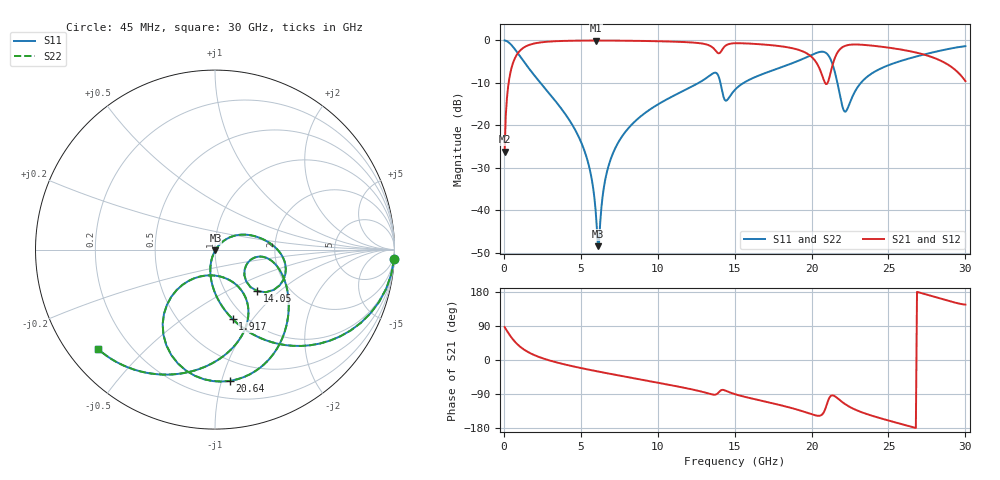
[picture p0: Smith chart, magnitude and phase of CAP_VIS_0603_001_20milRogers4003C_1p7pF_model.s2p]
! S-parameter model data by Modelithics Inc.  support@modelithics.com  813-866-6335  Tampa FL USA
! S-Parameter data specifications:
! Substrate: 20-mil Rogers 4003C, substrate thickness, H=0.508mm, Dielectric constant, Er=3.75
! PCB Mounting Pad Footprint: Pad width, PadW=0.90mm , Pad length, PadL=1.00mm , Pad gap, PadG (edge-to-edge)=1.00mm , Reference planes=3.0mm apart
! Created Wed Nov 18 13:18:57 2015
# hz S ma R 50
! 2 Port Network Data from SP1.SP block
! freq  magS11  angS11  magS21  angS21  magS12  angS12  magS22  angS22
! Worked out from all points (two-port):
!   401 points, 45 MHz to 30 GHz, reference 50 ohm
!   highest |S21| = -0.03 dB at 5.961 GHz (marker M1); lowest = -26.2 dB at 45 MHz (marker M2)
!   |S21| within 3 dB of the highest: 902.1 MHz to 13.95 GHz (13.05 GHz wide, 176 % of centre); 13.99 GHz to 19.68 GHz (5.691 GHz wide, 33.8 % of centre)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
!   lowest |S11| = -48.5 dB at 6.111 GHz (marker M3), VSWR 1.01, Z = 50.2 - j0.303 ohm
!   |S11| at or under -10 dB: 2.372 GHz to 12.67 GHz (10.29 GHz wide, 137 % of centre); 14.07 GHz to 15.59 GHz (1.516 GHz wide, 10.2 % of centre); 21.68 GHz to 23.21 GHz (1.529 GHz wide, 6.81 % of centre)
!   |S22| runs from -48.5 to 0.0 dB; largest |S21 - S12| = 0
!   S11 on the Smith chart (normalised r, x): 45 MHz: 1, -38; 1.917 GHz: 0.87, -0.80; 14.05 GHz: 1.40, -0.73; 20.64 GHz: 0.33, -1.06; 30 GHz: 0.09, -0.37
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4.5e7  0.9988 -3.0  0.04871 87.0  0.04871 87.0  0.9988 -3.0
2.696625e8  0.9596 -17.7  0.2809 72.3  0.2809 72.3  0.9596 -17.7
5.692125e8  0.8489 -34.7  0.5279 55.3  0.5279 55.3  0.8489 -34.7
1.917188e9  0.3998 -75.7  0.9147 14.0  0.9147 14.0  0.3998 -75.7
5.062462e9  0.0605 -108.8  0.9946 -21.7  0.9946 -21.7  0.0605 -108.8
5.661562e9  0.02574 -109.3  0.9959 -26.7  0.9959 -26.7  0.02574 -109.3
5.961112e9  0.009928 -99.1  0.996 -29.1  0.996 -29.1  0.009928 -99.1
6.110888e9  0.003756 -53.5  0.996 -30.3  0.996 -30.3  0.003756 -53.5
6.6351e9  0.02516 47.3  0.9955 -34.4  0.9955 -34.4  0.02516 47.3
7.2342e9  0.05354 46.8  0.9941 -39.0  0.9941 -39.0  0.05354 46.8
1.007992e10  0.1791 27.8  0.9775 -60.5  0.9775 -60.5  0.1791 27.8
1.352475e10  0.4016 -12.3  0.837 -90.7  0.837 -90.7  0.4016 -12.3
1.404896e10  0.3307 -44.4  0.7154 -81.8  0.7154 -81.8  0.3307 -44.4
1.44234e10  0.1944 -27.5  0.871 -81.1  0.871 -81.1  0.1944 -27.5
1.50225e10  0.2621 -8.6  0.9261 -90.2  0.9261 -90.2  0.2621 -8.6
2.003996e10  0.6779 -63.0  0.63 -143.6  0.63 -143.6  0.6779 -63.0
2.063906e10  0.7361 -83.6  0.4101 -145.3  0.4101 -145.3  0.7361 -83.6
2.138794e10  0.5071 -125.1  0.5303 -93.4  0.5303 -93.4  0.5071 -125.1
2.22117e10  0.1448 -89.8  0.867 -117.2  0.867 -117.2  0.1448 -89.8
2.505742e10  0.5148 -74.3  0.8196 -160.4  0.8196 -160.4  0.5148 -74.3
2.797804e10  0.7296 -107.9  0.6209 166.9  0.6209 166.9  0.7296 -107.9
3e10  0.8548 -139.5  0.3313 146.2  0.3313 146.2  0.8548 -139.5
